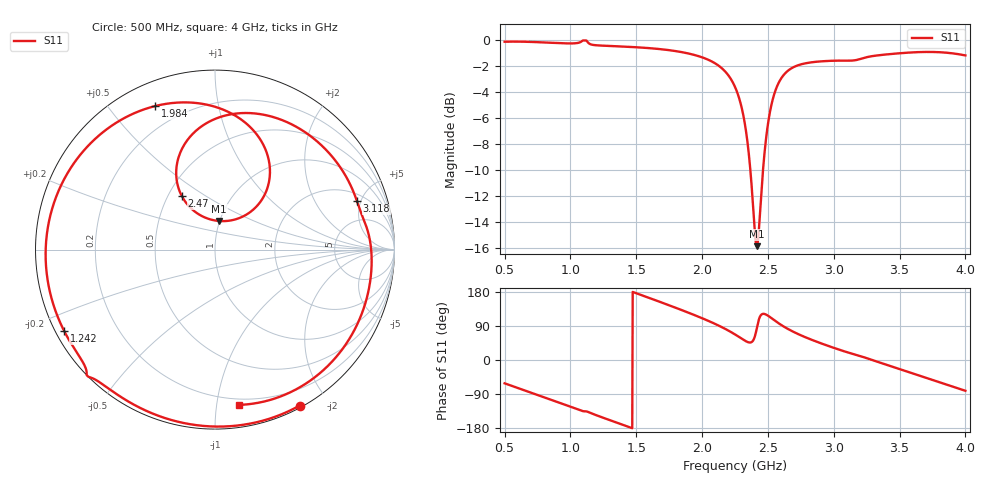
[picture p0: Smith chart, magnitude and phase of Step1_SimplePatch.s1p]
! TOUCHSTONE file generated by CST MICROWAVE STUDIO
! Date and time: Mon May 18 00:47:28 2020
! Project name: DualBand_DualMode_Antenna_FD_SteppedDesign.cst
! Parameters = {FPL=20; FPW=20; L=50; ST=10; SW=30; W=52; WF=7; ext=10; gap=1; inset=13}
! Header version: 2015
! Port assignment regex: !\s*Touchstone port\s*([0-9]+)\s*=\s*CST MWS port\s*([0-9]+)\s*\(\"(.*)\"\)(\s*mode\s*([0-9]+))?.*
! Touchstone port assignment:
! Touchstone port 1 = CST MWS port 1 ("")
# GHz S MA R 50
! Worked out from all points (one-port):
!   1006 points, 500 MHz to 4 GHz, reference 50 ohm
!   lowest |S11| = -15.9 dB at 2.414 GHz (marker M1), VSWR 1.38, Z = 49.6 + j16.2 ohm
!   |S11| at or under -10 dB: 2.367 GHz to 2.463 GHz (96.07 MHz wide, 3.98 % of centre)
!   S11 on the Smith chart (normalised r, x): 500 MHz: 0.02, -1.68; 1.242 GHz: 0.02, -0.25; 1.984 GHz: 0.10, +0.66; 2.47 GHz: 0.59, +0.40; 3.118 GHz: 2.60, +4.64; 4 GHz: 0.16, -1.15
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0.5  0.9886 -61.5
0.717  0.9865 -88.2
0.9375  0.9756 -115.3
1.088  0.9949 -134.3
1.1265  0.9916 -136.1
1.242  0.955 -151.6
1.375  0.9485 -168.2
1.592  0.9347 164.6
1.8125  0.9076 136.1
1.984  0.8664 112.6
2.131  0.7957 90.0
2.25  0.6621 67.5
2.299  0.5552 56.7
2.3375  0.4329 48.7
2.4005  0.184 61.9
2.4145  0.161 82.1
2.4355  0.1998 111.1
2.4705  0.3517 121.8
2.516  0.5315 113.2
2.5755  0.6763 98.3
2.6875  0.7856 75.5
2.894  0.8299 45.2
3.118  0.8358 18.8
3.125  0.8359 18.1
3.342  0.8769 -5.8
3.5625  0.8973 -31.1
3.797  0.9012 -58.0
4  0.8756 -81.2
